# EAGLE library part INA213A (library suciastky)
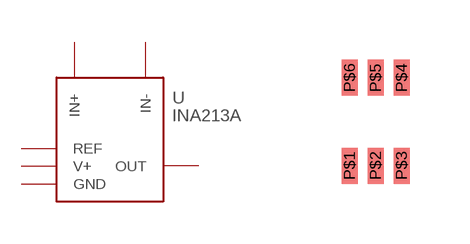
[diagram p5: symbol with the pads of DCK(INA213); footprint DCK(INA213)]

Designator prefix -

## INA213A  [DCK(INA213)]
P$1  REF
P$2  GND  pwr
P$3  V+  out
P$4  IN+  in
P$5  IN-  in
P$6  OUT  out

## Footprint DCK(INA213) (pad centres in mm)
smd 0.4 x 0.9: P$1 -0.65,-1.1; P$2 0,-1.1; P$3 0.65,-1.1; P$4 0.65,1.1; P$5 0,1.1; P$6 -0.65,1.1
